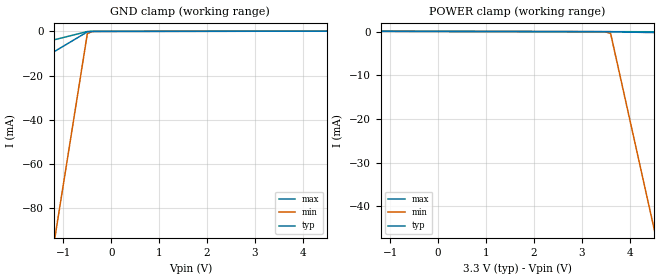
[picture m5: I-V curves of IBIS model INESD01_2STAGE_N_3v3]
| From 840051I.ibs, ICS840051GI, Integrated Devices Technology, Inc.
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[Model] INESD01_2STAGE_N_3v3
Model_type   Input
Polarity   Non-Inverting
Vinl = 0.8V
Vinh = 2.0V
|   typ   min   max
C_comp   2pF   1.5pF   2.5pF
|   typ   min   max
[Voltage range]  3.3V   3.15V   3.45V
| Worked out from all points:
|   GND clamp passes 1 mA (typ) near -0.56 V on its own axis
[GND_clamp]
|Voltage   I(typ)   I(min)   I(max)
-3.3V     -36.4mA    -382.1mA   -15.22mA
-1.2V     -9.271mA   -96.28mA   -3.853mA
-1.1V     -7.979mA   -82.66mA   -3.312mA
-500mV    -227.8uA   -989.9uA   -65.11uA
-400mV    -30.81uA   -105.6uA   -11.01uA
-300mV    -7.585uA   -16.23uA   -6.189uA
6.6V      129.3uA    124.7uA    134.2uA
[POWER_clamp]
|Voltage   I(typ)   I(min)   I(max)
-3.3V     129.3uA    121.5uA    137.6uA
3.4V      -1.963uA   -9.687uA   1.322uA
3.5V      -4.012uA   -52.24uA   -711.7nA
3.6V      -7.585uA   -433.5uA   -2.745uA
4.5V      -216.6uA   -44.85mA   -21.11uA
4.6V      -239.9uA   -49.78mA   -23.15uA
6.6V      -704.4uA   -148.5mA   -63.97uA
